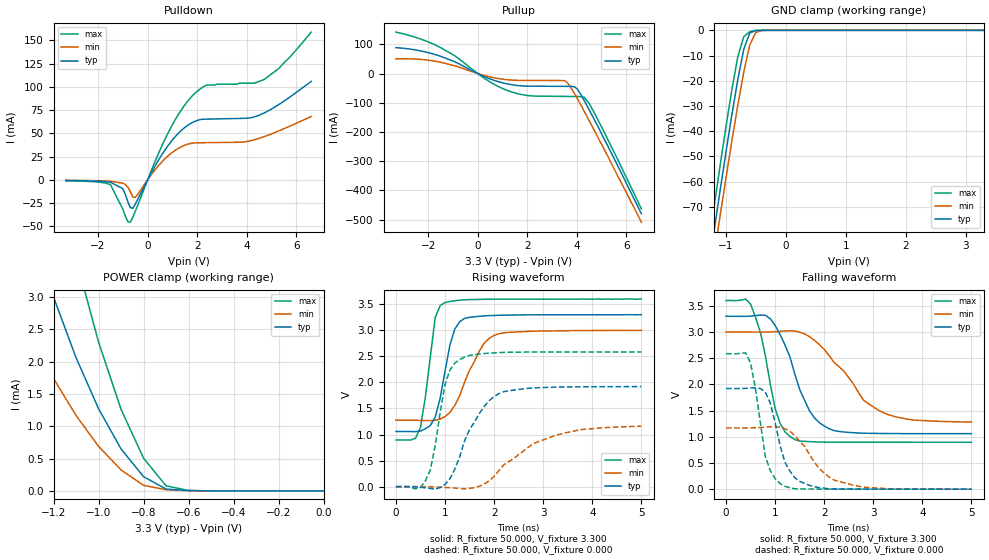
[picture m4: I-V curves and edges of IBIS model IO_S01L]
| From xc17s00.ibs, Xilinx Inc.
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|   Model IO_S01L
[Model]   IO_S01L
Model_type   I/O
Polarity   Non-Inverting
Enable   Active-High
Vinl =   0.800V
Vinh =   2.000V
Vmeas =   1.650V
Cref =  50.000pF
Rref =   1.000M
Vref =  0.000V
C_comp   2.750pF   2.250pF   3.250pF
[Temperature Range]   50.000   100.000   0.000
[Voltage Range]   3.300V   3.000V   3.600V
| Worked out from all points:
|   slope of the pulldown table from 0 to 0.495 V, typ, clamps not added: 20.8 ohm
|   slope of the pullup table from 0 to 0.495 V, typ, clamps not added: 27 ohm
|   GND clamp passes 1 mA (typ) near -0.60 V on its own axis
|   POWER clamp passes 1 mA (typ) near -0.96 V on its own axis
|   rising waveform, R_fixture 50.000, V_fixture 3.300: 20-80 % time 295ps typ, 502ps min, 225ps max; typ from 1.06 V to 3.3 V
|   rising waveform, R_fixture 50.000, V_fixture 0.000: 20-80 % time 575ps typ, 1.05ns min, 297ps max; typ from 0 V to 1.92 V
|   falling waveform, R_fixture 50.000, V_fixture 3.300: 20-80 % time 543ps typ, 897ps min, 359ps max; typ from 3.3 V to 1.06 V
|   falling waveform, R_fixture 50.000, V_fixture 0.000: 20-80 % time 348ps typ, 613ps min, 271ps max; typ from 1.92 V to 0 V
[Pulldown]
| voltage   I(typ)   I(min)   I(max)
-3.3V     -600uA     -400uA     -1mA
-1.5V     -2.5mA     -1.5mA     -5mA
-1V       -9.44mA    -3.56mA    -31.42mA
-800mV    -23.41mA   -7.59mA    -44.81mA
-700mV    -29.72mA   -12.65mA   -45.51mA
-500mV    -26.19mA   -18.96mA   -34.02mA
700mV     32.2mA     22.71mA    43.69mA
1.8V      61.63mA    39.51mA    90.28mA
2.4V      65.36mA    40.06mA    102mA
4.7V      71.97mA    46.5mA     108mA
5.3V      81.16mA    52.79mA    120mA
6.6V      106mA      68.14mA    159mA
[Pullup]
| voltage   I(typ)   I(min)   I(max)
-3.3V     88.66mA    50.5mA     142mA
-1.5V     59.21mA    38.72mA    89.11mA
-900mV    39.17mA    25.89mA    59mA
400mV     -15.21mA   -9.642mA   -23.79mA
1.2V      -35.64mA   -21.22mA   -58.08mA
2.1V      -43.2mA    -23.48mA   -76.02mA
3.6V      -43.97mA   -29.75mA   -78.34mA
4V        -51.68mA   -83.1mA    -78.68mA
4.3V      -93.08mA   -130mA     -81.45mA
4.5V      -125mA     -162mA     -103mA
5.1V      -224mA     -259mA     -200mA
6.6V      -480mA     -509mA     -463mA
[GND_clamp]
| voltage   I(typ)   I(min)   I(max)
-3.3V     -434mA     -434mA     -435mA
-1.3V     -96.3mA    -106mA     -87.19mA
-1.2V     -80.19mA   -89.89mA   -70.7mA
-1.1V     -64.31mA   -74.33mA   -54.49mA
-1V       -48.75mA   -59.03mA   -38.71mA
-900mV    -33.69mA   -44.1mA    -23.71mA
-800mV    -19.54mA   -29.76mA   -10.47mA
-700mV    -7.504mA   -16.51mA   -2.514mA
-600mV    -1.037mA   -5.805mA   -545uA
-500mV    -70.45uA   -808uA     -33.21uA
-400mV    -3.698uA   -72.41uA   -2.036uA
3.3V      204pA      39.97nA    67.46pA
[POWER_clamp]
| voltage   I(typ)   I(min)   I(max)
-3.3V     38.24mA    23.14mA    61.44mA
-1.4V     5.246mA    3.126mA    8.7mA
-1.3V     4.067mA    2.398mA    6.818mA
-1.2V     3.001mA    1.742mA    5.11mA
-1.1V     2.064mA    1.169mA    3.598mA
-1V       1.274mA    691uA      2.306mA
-900mV    651uA      325uA      1.264mA
-800mV    221uA      87.03uA    508uA
-700mV    28.94uA    18.03uA    79.19uA
-600mV    5.041uA    4.415uA    6.917uA
0V        204pA      1.705nA    79.84pA
[Ramp]
| variable   typ   min   max
dV/dt_r   1.152/0.573n   0.695/1.045n   1.551/0.280n
dV/dt_f   1.345/0.540n   1.031/0.916n   1.623/0.342n
R_load = 50.000
[Rising Waveform]
R_fixture = 50.000
V_fixture = 3.300
V_fixture_min = 3.000
V_fixture_max = 3.600
L_fixture = 0.000H
C_fixture = 0.000F
| time   V(typ)   V(min)   V(max)
0s        1.059V     1.275V     895mV
400ps     1.055V     1.275V     928mV
500ps     1.067V     1.271V     1.136V
800ps     1.334V     1.274V     3.242V
1ns       2.212V     1.343V     3.533V
1.1ns     2.716V     1.424V     3.555V
1.3ns     3.166V     1.746V     3.578V
1.7ns     3.27V      2.604V     3.594V
2ns       3.285V     2.902V     3.598V
5ns       3.3V       2.999V     3.6V
[Rising Waveform]
R_fixture = 50.000
V_fixture = 0.000
V_fixture_min = 0.000
V_fixture_max = 0.000
L_fixture = 0.000H
C_fixture = 0.000F
| time   V(typ)   V(min)   V(max)
0s        0V         0V         0V
600ps     -23.15mV   -251uV     110mV
700ps     -34.32mV   -2.234mV   321mV
1ns       42.35mV    -15.78mV   1.959V
1.3ns     578mV      -35.37mV   2.439V
1.5ns     1.096V     -33.89mV   2.517V
1.8ns     1.543V     50.44mV    2.554V
2.2ns     1.824V     419mV      2.576V
3.3ns     1.91V      995mV      2.584V
5ns       1.92V      1.159V     2.585V
[Falling Waveform]
R_fixture = 50.000
V_fixture = 3.300
V_fixture_min = 3.000
V_fixture_max = 3.600
L_fixture = 0.000H
C_fixture = 0.000F
| time   V(typ)   V(min)   V(max)
0s        3.3V       3V         3.6V
500ps     3.302V     2.998V     3.53V
700ps     3.323V     2.997V     2.995V
1ns       3.126V     3.005V     1.538V
1.2ns     2.752V     3.019V     1.096V
1.4ns     2.201V     3.018V     947mV
1.7ns     1.495V     2.91V      907mV
2.2ns     1.118V     2.42V      897mV
3.2ns     1.062V     1.461V     896mV
5ns       1.059V     1.282V     895mV
[Falling Waveform]
R_fixture = 50.000
V_fixture = 0.000
V_fixture_min = 0.000
V_fixture_max = 0.000
L_fixture = 0.000H
C_fixture = 0.000F
| time   V(typ)   V(min)   V(max)
0s        1.921V     1.169V     2.585V
400ps     1.924V     1.168V     2.602V
500ps     1.931V     1.17V      2.405V
600ps     1.933V     1.173V     1.917V
800ps     1.853V     1.184V     626mV
1ns       1.273V     1.193V     201mV
1.2ns     516mV      1.154V     54.62mV
1.5ns     147mV      916mV      5.838mV
2.2ns     5.607mV    174mV      571uV
5ns       270uV      455uV      69.19uV
